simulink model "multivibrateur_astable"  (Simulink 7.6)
settings: Solver=ode15s  StartTime=0.0  StopTime=1  MaxStep=1e-6  RelTol=1e-3
StopFcn:
  | close all, clc
  | load schmidt.mat
  | plot(x(1,:),x(2,:),'--',x(1,:),x(3,:))
  | title('Multivibrateur astable à amplificateur opérationnel')
  | xlabel('temps')
  | grid
libraries: fl_lib x11, nesl_utility x4, elec_lib x1

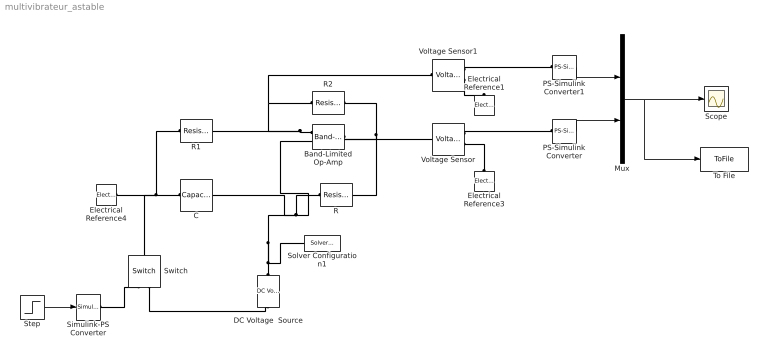
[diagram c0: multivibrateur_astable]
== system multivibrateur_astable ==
  Band-Limited Op-Amp : elec_lib/Integrated Circuits/Band-Limited Op-Amp  DialogController=NetworkEngine.DynNeDlgSource  SystemSampleTime=-1  A=1000  Rin=1e+06 Ohm  Rout=100 Ohm  Vmin=-15 V  Vmax=15 V  Vdotmax=1000 V/s  f=1e+05 Hz  V0=0 V  LocalVarNames=|power  LocalVarDescs=|Dissipated power (W)  LocalVarLogging=0
  C : fl_lib/Electrical/Electrical Elements/Capacitor  DialogController=NetworkEngine.DynNeDlgSource  SystemSampleTime=-1  c=1e-3 F  v0=0 V  r=1e-12 Ohm  g=0 1/Ohm  i_Log=off  v_Log=off  vc_Log=off  LocalVarNames=|current|voltage|power  LocalVarDescs=|Capacitor current (A)|Voltage across capacitor (V)|Power (W)  LocalVarLogging=[0 0 0]
  DC Voltage  Source : fl_lib/Electrical/Electrical Sources/DC Voltage Source  DialogController=NetworkEngine.DynNeDlgSource  SystemSampleTime=-1  v0=1 V  i_Log=off  v_Log=off  LocalVarNames=|i|v  LocalVarDescs=|i|v  LocalVarLogging=[0 0]
  Electrical Reference1 : fl_lib/Electrical/Electrical Elements/Electrical Reference  DialogController=NetworkEngine.DynNeDlgSource  SystemSampleTime=-1  i_Log=off  LocalVarNames=|i  LocalVarDescs=|i  LocalVarLogging=[]
  Electrical Reference3 : fl_lib/Electrical/Electrical Elements/Electrical Reference  DialogController=NetworkEngine.DynNeDlgSource  SystemSampleTime=-1  i_Log=off  LocalVarNames=|i  LocalVarDescs=|i  LocalVarLogging=[]
  Electrical Reference4 : fl_lib/Electrical/Electrical Elements/Electrical Reference  DialogController=NetworkEngine.DynNeDlgSource  SystemSampleTime=-1  i_Log=off  LocalVarNames=|i  LocalVarDescs=|i  LocalVarLogging=[]
  Mux : Mux  Inputs=2
  PS-Simulink Converter : nesl_utility/PS-Simulink Converter  DialogController=NetworkEngine.DynNeUtilDlgSource  SystemSampleTime=-1  PhysicalDomain=network_engine_domain  LeftPortType=input  RightPortType=output  SubClassName=ps_output  Unit=1  AffineConversion=off
  PS-Simulink Converter1 : nesl_utility/PS-Simulink Converter  DialogController=NetworkEngine.DynNeUtilDlgSource  SystemSampleTime=-1  PhysicalDomain=network_engine_domain  LeftPortType=input  RightPortType=output  SubClassName=ps_output  Unit=1  AffineConversion=off
  R : fl_lib/Electrical/Electrical Elements/Resistor  DialogController=NetworkEngine.DynNeDlgSource  SystemSampleTime=-1  R=1e3 Ohm  i_Log=off  v_Log=off  LocalVarNames=|current|voltage|power  LocalVarDescs=|Resistor current (A)|Voltage across resistor (V)|Power (W)  LocalVarLogging=[0 0 0]
  R1 : fl_lib/Electrical/Electrical Elements/Resistor  DialogController=NetworkEngine.DynNeDlgSource  SystemSampleTime=-1  R=1 kOhm  i_Log=off  v_Log=off  LocalVarNames=|current|voltage|power  LocalVarDescs=|Resistor current (A)|Voltage across resistor (V)|Power (W)  LocalVarLogging=[0 0 0]
  R2 : fl_lib/Electrical/Electrical Elements/Resistor  DialogController=NetworkEngine.DynNeDlgSource  SystemSampleTime=-1  R=10e3 Ohm  i_Log=off  v_Log=off  LocalVarNames=|current|voltage|power  LocalVarDescs=|Resistor current (A)|Voltage across resistor (V)|Power (W)  LocalVarLogging=[0 0 0]
  Scope : Scope
  Simulink-PS Converter : nesl_utility/Simulink-PS Converter  DialogController=NetworkEngine.DynNeUtilDlgSource  SystemSampleTime=-1  PhysicalDomain=network_engine_domain  LeftPortType=input  RightPortType=output  SubClassName=ps_input  Unit=1  AffineConversion=off  InputFilterTimeConstant=.001  UdotUserProvided=0
  Solver Configuration1 : nesl_utility/Solver Configuration  DialogController=NetworkEngine.DynNeUtilDlgSource  SystemSampleTime=-1  PhysicalDomain=network_engine_domain  LeftPortType=input  RightPortType=generic  SubClassName=solver  Accelerate=off  Profile=off  ResidualTolerance=1e-40  MaxNonlinIter=12  MaxModeIter=2  DoFixedCost=off  UseLocalSampling=off  DoDC=on  LinearAlgebra=Full  LocalSolverSampleTime=.001  LocalSolverChoice=NE_BACKWARD_EULER_ADVANCER  UseLocalSolver=off
  Step : Step  Time=0.1  Before=1  After=0  SampleTime=0
  Switch : fl_lib/Electrical/Electrical Elements/Switch  DialogController=NetworkEngine.DynNeDlgSource  SystemSampleTime=-1  R_closed=0.01 Ohm  G_open=1e-08 1/Ohm  Threshold=0  i_Log=off  v_Log=off  LocalVarNames=|i|v  LocalVarDescs=|i|v  LocalVarLogging=[0 0]
  To File : ToFile  Filename=schmidt  MatrixName=x
  Voltage Sensor : fl_lib/Electrical/Electrical Sensors/Voltage Sensor  DialogController=NetworkEngine.DynNeDlgSource  SystemSampleTime=-1  i1_Log=off  v1_Log=off  LocalVarNames=|i1|v1  LocalVarDescs=|i1|v1  LocalVarLogging=[]
  Voltage Sensor1 : fl_lib/Electrical/Electrical Sensors/Voltage Sensor  DialogController=NetworkEngine.DynNeDlgSource  SystemSampleTime=-1  i1_Log=off  v1_Log=off  LocalVarNames=|i1|v1  LocalVarDescs=|i1|v1  LocalVarLogging=[]
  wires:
  Step/1 -> Simulink-PS Converter/1
  Mux/1 -> Scope/1, To File/1
  PS-Simulink Converter/1 -> Mux/2
  PS-Simulink Converter1/1 -> Mux/1
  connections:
  R1/LConn1 -- Switch/LConn1 -- C/LConn1 -- Electrical Reference4/LConn1
  Simulink-PS Converter/RConn1 -- Switch/RConn1
  Electrical Reference3/LConn1 -- Voltage Sensor/RConn2
  Switch/RConn2 -- DC Voltage  Source/RConn1
  Voltage Sensor/RConn1 -- PS-Simulink Converter/LConn1
  Band-Limited Op-Amp/LConn1 -- R2/LConn1 -- Voltage Sensor1/LConn1 -- R1/RConn1
  R2/RConn1 -- Band-Limited Op-Amp/RConn1 -- Voltage Sensor/LConn1 -- R/RConn1
  DC Voltage  Source/LConn1 -- Solver Configuration1/RConn1 -- Band-Limited Op-Amp/LConn2 -- C/RConn1 -- R/LConn1
  Voltage Sensor1/RConn1 -- PS-Simulink Converter1/LConn1
  Voltage Sensor1/RConn2 -- Electrical Reference1/LConn1
